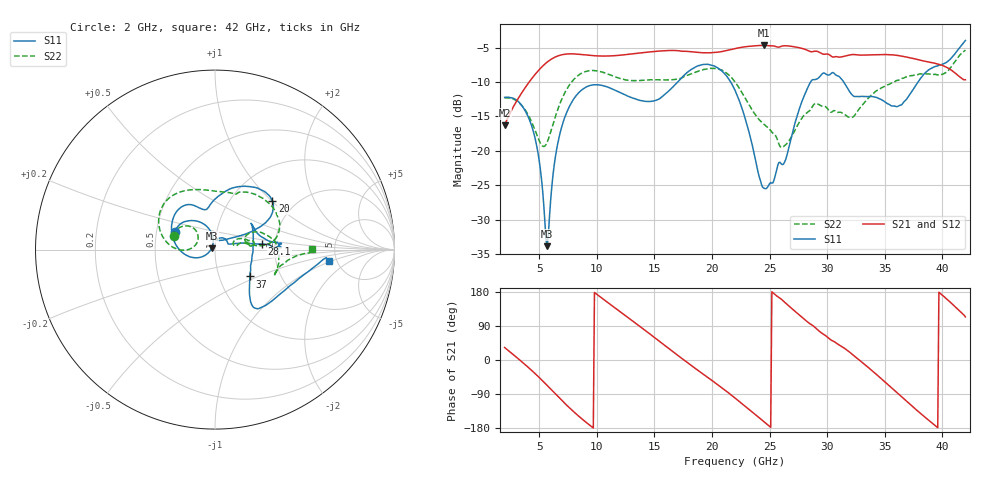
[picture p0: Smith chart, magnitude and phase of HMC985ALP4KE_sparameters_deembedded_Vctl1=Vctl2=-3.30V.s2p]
!s2p File: Measurements: S11, S21, S12, S22
# GHz S dB R 50.0
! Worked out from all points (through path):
!   401 points, 2 GHz to 42 GHz, reference 50 ohm
!   highest |S21| = -4.66 dB at 24.5 GHz (marker M1); lowest = -16.3 dB at 2 GHz (marker M2)
!   lowest |S11| = -33.9 dB at 5.7 GHz (marker M3), VSWR 1.04, Z = 48.1 + j0.655 ohm
!   |S11| at or under -10 dB: start of sweep to 17.01 GHz; 21.63 GHz to 28.55 GHz (6.922 GHz wide, 27.6 % of centre); 31.45 GHz to 37.88 GHz (6.436 GHz wide, 18.6 % of centre)
!   |S22| runs from -19.5 to -5.3 dB; largest |S21 - S12| = 0.00073
!   S11 on the Smith chart (normalised r, x): 2 GHz: 0.62, +0.13; 20 GHz: 1.54, +1.01; 28.1 GHz: 1.70, +0.11; 37 GHz: 1.40, -0.45; 42 GHz: 4.30, -0.89
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2  -12.21 156.7  -16.28 32.9  -16.29 32.9  -12.30 161.4
4.4  -16.64 111.7  -9.39 -28.9  -9.39 -28.9  -16.00 134.8
5  -21.38 100.8  -8.19 -46.1  -8.19 -46.1  -18.50 142.4
5.7  -33.88 160.4  -7.08 -67.4  -7.08 -67.4  -18.72 170.2
6.8  -17.51 -160.9  -6.09 -101.6  -6.09 -101.6  -13.14 178.4
8.7  -11.13 150.3  -5.99 -155.1  -5.99 -155.1  -8.68 147.3
10.5  -10.49 124.2  -6.20 162.0  -6.20 162.0  -8.55 120.2
12.6  -11.96 111.6  -5.99 114.6  -5.99 114.6  -9.70 91.9
15.4  -12.46 98.8  -5.48 50.3  -5.48 50.3  -9.66 70.8
17.6  -8.97 74.3  -5.51 -0.6  -5.51 -0.6  -9.17 67.0
20  -7.56 40.3  -5.72 -54.0  -5.72 -54.0  -7.99 34.8
22  -11.18 26.7  -5.12 -100.4  -5.12 -100.4  -9.96 7.4
24.5  -25.43 72.9  -4.66 -162.4  -4.66 -162.4  -16.11 14.2
26.1  -22.00 25.7  -4.74 158.4  -4.74 158.3  -19.49 18.4
28.1  -11.62 6.7  -5.24 105.3  -5.24 105.3  -14.66 17.3
28.7  -9.68 1.2  -5.57 92.0  -5.57 91.9  -13.61 14.4
30.6  -8.69 4.5  -6.34 48.6  -6.34 48.6  -14.13 10.6
32.4  -12.10 24.8  -5.99 9.3  -5.99 9.3  -14.79 22.7
35.4  -13.26 10.3  -6.00 -68.3  -6.00 -68.4  -10.30 14.3
37  -12.22 -37.7  -6.38 -111.7  -6.38 -111.7  -9.18 3.2
39.5  -7.69 -51.2  -7.31 -176.1  -7.32 -176.2  -8.90 -23.1
42  -3.93 -5.6  -9.64 113.7  -9.65 113.6  -5.33 0.4
